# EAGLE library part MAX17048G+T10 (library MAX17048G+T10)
3A 1-Cell/2-Cell Fuel Gauge with ModelGauge Source: Datasheet
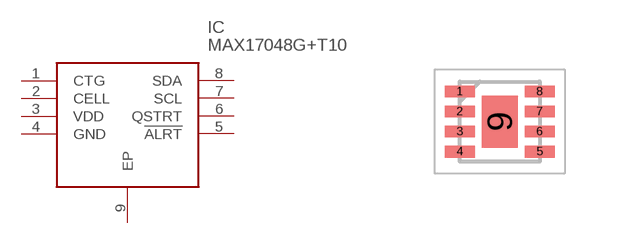
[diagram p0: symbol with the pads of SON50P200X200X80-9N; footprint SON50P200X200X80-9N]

Designator prefix IC

## MAX17048G+T10 (Arrow_Part_Number: MAX17048G+T10; Arrow_Price-Stock: https://www.arrow.com/en/products/max17048gt10/analog-devices?utm_currency=USD&region=nac; Description: 3A 1-Cell/2-Cell Fuel Gauge with ModelGauge; Height: 0.8mm; Manufacturer_Name: Analog Devices; Manufacturer_Part_Number: MAX17048G+T10; Mouser_Part_Number: 700-MAX17048G+T10; Mouser_Price-Stock: https://www.mouser.co.uk/ProductDetail/Analog-Devices-Maxim-Integrated/MAX17048G%2bT10?qs=D7PJwyCwLAoGnnn8jEPRBQ%3D%3D)  [SON50P200X200X80-9N]
1  CTG
2  CELL
3  VDD
4  GND
5  !ALRT
6  QSTRT
7  SCL
8  SDA
9  EP

## Footprint SON50P200X200X80-9N (pad centres in mm)
T822+3
smd 0.75 x 0.3: 1 -1,0.75; 2 -1,0.25; 3 -1,-0.25; 4 -1,-0.75; 5 1,-0.75; 6 1,-0.25; 7 1,0.25; 8 1,0.75
smd 0.9 x 1.3: 9 0,0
